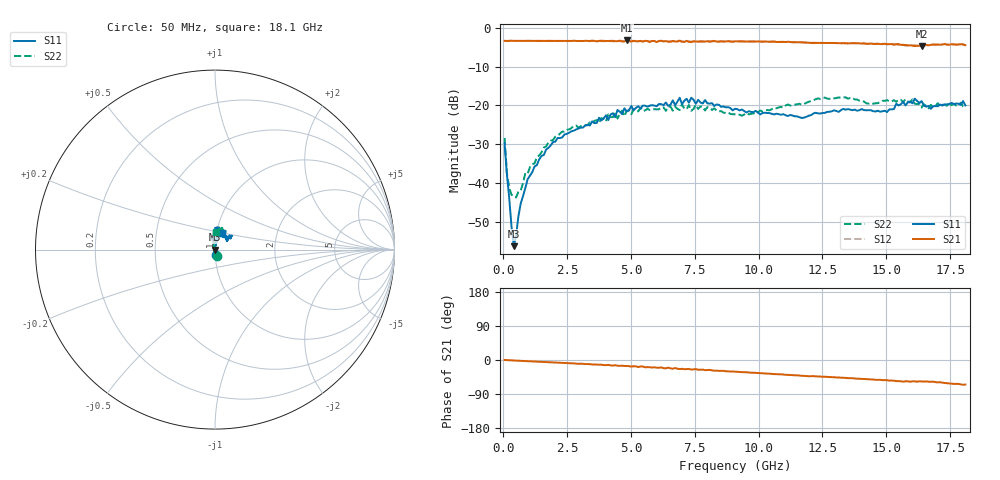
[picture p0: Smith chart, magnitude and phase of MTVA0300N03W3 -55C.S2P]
! Network Analyzer HP8720D.06.14 Serial No. US36140669
!  7 Jul 2005  08:21:51
! Frequency  S11  S21  S12  S22
# HZ  S  DB R 50
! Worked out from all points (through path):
!   201 points, 50 MHz to 18.1 GHz, reference 50 ohm
!   highest |S21| = -3.32 dB at 4.833 GHz (marker M1); lowest = -4.8 dB at 16.39 GHz (marker M2)
!   group delay of S21, straight-line fit = 9.96 ps
!   lowest |S11| = -56.1 dB at 411 MHz (marker M3), VSWR 1.00, Z = 49.8 - j0.0426 ohm
!   |S11| at or under -10 dB: start of sweep to end of sweep
!   |S22| runs from -43.6 to -17.9 dB; largest |S21 - S12| = 0.023
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5e7  -29.72 -83.5  -3.41 0.0  -3.42 0.1  -28.33 -74.5
1.4025e8  -37.75 -86.3  -3.45 -0.3  -3.44 -0.3  -37.39 -107.2
2.305e8  -43.76 -89.5  -3.42 -0.6  -3.42 -0.6  -41.12 -132.2
4.11e8  -56.09 -164.2  -3.42 -1.3  -3.42 -1.3  -43.36 -173.0
6.8175e8  -45.13 110.4  -3.42 -2.2  -3.42 -2.2  -41.83 141.7
8.6225e8  -41.17 90.0  -3.41 -2.7  -3.43 -2.8  -37.36 134.3
1.22325e9  -35.66 88.4  -3.42 -3.9  -3.43 -4.0  -34.86 112.6
2.0355e9  -29.28 81.0  -3.42 -6.6  -3.43 -6.7  -28.02 102.8
3.1185e9  -25.67 81.1  -3.45 -10.0  -3.48 -10.3  -24.95 104.4
4.83325e9  -21.54 83.2  -3.32 -15.7  -3.43 -16.5  -21.35 90.3
6.09675e9  -19.61 80.6  -3.47 -20.4  -3.40 -20.3  -20.97 88.8
6.909e9  -18.02 84.8  -3.36 -23.9  -3.48 -23.0  -21.17 80.3
6.99925e9  -19.67 83.8  -3.62 -23.2  -3.68 -24.6  -19.66 81.6
7.36025e9  -18.01 78.7  -3.75 -25.2  -3.58 -24.4  -21.36 85.9
7.54075e9  -19.56 79.8  -3.59 -24.0  -3.45 -25.8  -19.82 86.4
9.075e9  -20.84 93.8  -3.55 -30.7  -3.54 -30.8  -22.26 73.9
1.21435e10  -22.07 70.4  -3.94 -42.6  -3.90 -42.7  -18.70 73.7
1.512175e10  -21.00 38.6  -4.28 -54.4  -4.14 -54.0  -18.94 73.2
1.602425e10  -19.45 40.7  -4.58 -56.3  -4.75 -58.0  -18.43 60.4
1.638525e10  -18.86 38.3  -4.79 -56.5  -4.60 -56.1  -20.53 65.1
1.674625e10  -20.85 51.4  -4.42 -57.6  -4.53 -58.1  -19.83 73.8
1.81e10  -19.99 65.7  -4.52 -64.8  -4.62 -65.8  -20.23 85.8
